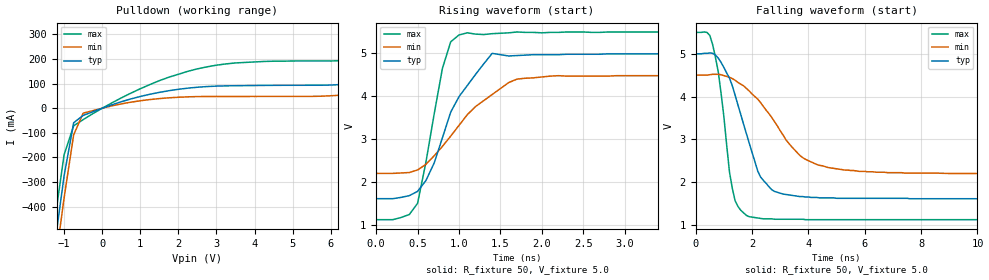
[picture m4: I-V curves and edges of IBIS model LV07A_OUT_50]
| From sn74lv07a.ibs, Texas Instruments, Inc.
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|   Model LV07A_OUT_50
[Model]   LV07A_OUT_50
Model_type  Open_drain
Polarity   Non-Inverting
Vmeas = 2.50v
Cref = 15pf
| variable   typ   min   max
C_comp   4.62pf   3.47pf   5.77pf
[Temperature Range]   25   85   -40
[Voltage Range]   5.0   4.5   5.5
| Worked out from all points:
|   slope of the pulldown table from 0 to 0.75 V, typ, clamps not added: 19.9 ohm
|   falling waveform, R_fixture 50, V_fixture 5.0: 20-80 % time 927ps typ, 1.61ns min, 475ps max; typ from 5 V to 1.61 V
|   rising waveform, R_fixture 50, V_fixture 5.0: 20-80 % time 465ps typ, 677ps min, 245ps max; typ from 1.61 V to 5 V
[Pulldown]
|   Voltage   I(typ)   I(min)   I(max)
-5V       -5.14A     -5.22A     -5.05A
-1.5V     -853mA     -945mA     -756mA
-1.25V    -557mA     -649mA     -461mA
-1V       -274mA     -363mA     -188mA
-750mV    -58.9mA    -108mA     -71.3mA
-500mV    -29.2mA    -20mA      -46.2mA
0V        -3.33nA    -3.4nA     -3.57nA
1.25V     56.7mA     35.2mA     96mA
2.5V      85.3mA     47.3mA     160mA
3.5V      91.4mA     47.8mA     184mA
6.75V     103mA      58.5mA     199mA
10V       179mA      107mA      329mA
[Ramp]
| variable   typ   min   max
dV/dt_r   2.15E+00/8.50E-10   1.50E+00/1.76E-09   2.72E+00/3.42E-10
dV/dt_f   2.05E+00/9.19E-10   1.39E+00/1.59E-09   2.64E+00/5.26E-10
R_load = 50
[Falling Waveform]
R_fixture = 50
V_fixture = 5.0
V_fixture_min = 4.5
V_fixture_max = 5.5
|   Time   V(typ)   V(min)   V(max)
0s        5V         4.5V       5.5V
600ps     5.01V      4.52V      5.22V
800ps     4.9V       4.52V      4.58V
1.3ns     4.25V      4.42V      1.85V
1.9ns     2.91V      4.13V      1.19V
2.3ns     2.12V      3.86V      1.15V
2.8ns     1.78V      3.41V      1.13V
3.8ns     1.66V      2.57V      1.13V
5.3ns     1.62V      2.28V      1.12V
25ns      1.61V      2.2V       1.12V
[Rising Waveform]
R_fixture = 50
V_fixture = 5.0
V_fixture_min = 4.5
V_fixture_max = 5.5
|   Time   V(typ)   V(min)   V(max)
0s        1.61V      2.2V       1.12V
400ps     1.68V      2.22V      1.24V
500ps     1.78V      2.28V      1.5V
800ps     3.03V      2.83V      4.65V
900ps     3.63V      3.07V      5.27V
1.1ns     4.25V      3.57V      5.48V
1.4ns     5V         4.04V      5.46V
1.7ns     4.95V      4.4V       5.5V
2.2ns     4.97V      4.48V      5.49V
25ns      5V         4.5V       5.5V
